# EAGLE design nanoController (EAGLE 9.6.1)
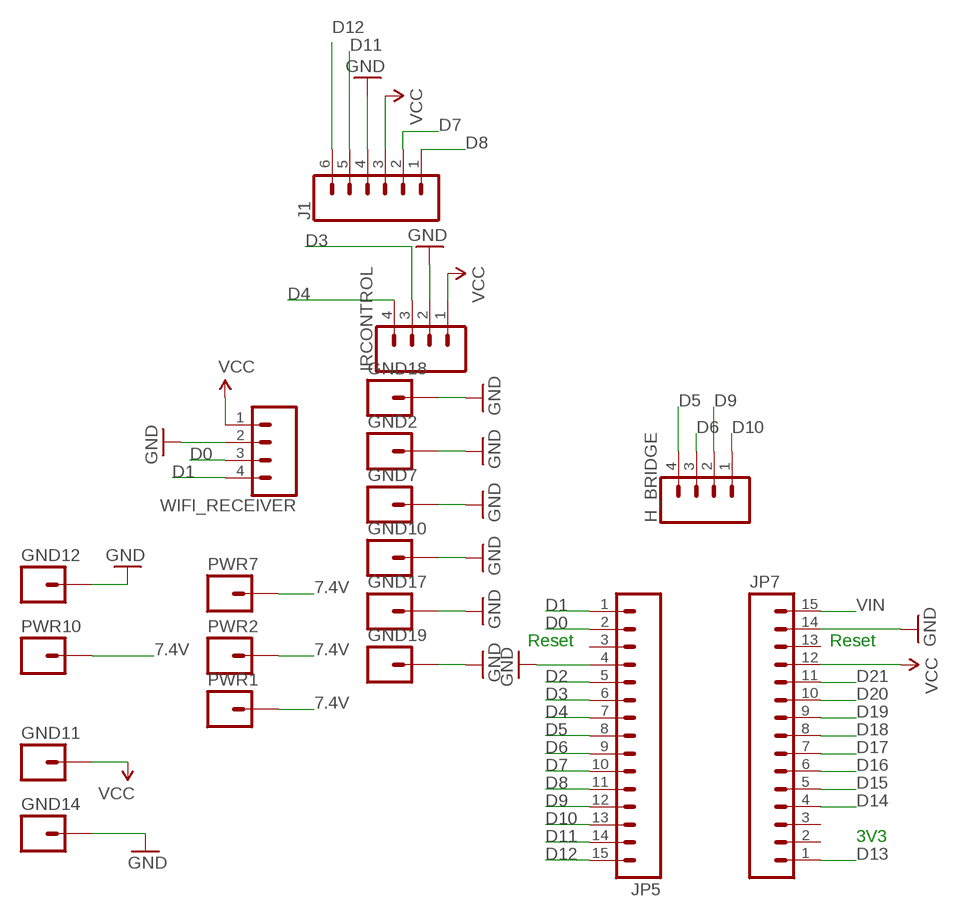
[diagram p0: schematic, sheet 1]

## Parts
GND2  M01PTH_LONGPAD  [1X01_LONGPAD]
GND7  M01PTH_LONGPAD  [1X01_LONGPAD]
GND10  M01PTH_LONGPAD  [1X01_LONGPAD]
GND11  M01PTH_LONGPAD  [1X01_LONGPAD]
GND12  M01PTH_LONGPAD  [1X01_LONGPAD]
GND14  M01PTH_LONGPAD  [1X01_LONGPAD]
GND17  M01PTH_LONGPAD  [1X01_LONGPAD]
GND18  M01PTH_LONGPAD  [1X01_LONGPAD]
GND19  M01PTH_LONGPAD  [1X01_LONGPAD]
H_BRIDGE  CONN_04LONGPADS  [1X04_LONGPADS]
IRCONTROL  CONN_04LONGPADS  [1X04_LONGPADS]
J1  CONN_06SILK_FEMALE_PTH  [1X06]
JP5  M15  [1X15]
JP7  M15  [1X15]
PWR1  M01PTH_LONGPAD  [1X01_LONGPAD]
PWR2  M01PTH_LONGPAD  [1X01_LONGPAD]
PWR7  M01PTH_LONGPAD  [1X01_LONGPAD]
PWR10  M01PTH_LONGPAD  [1X01_LONGPAD]
WIFI_RECEIVER  CONN_04LONGPADS  [1X04_LONGPADS]

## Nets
7.4V: PWR1.1 PWR2.1 PWR7.1 PWR10.1
D0: JP5.2 WIFI_RECEIVER.3
D1: JP5.1 WIFI_RECEIVER.4
D2: JP5.5
D3: IRCONTROL.3 JP5.6
D4: IRCONTROL.4 JP5.7
D5: H_BRIDGE.4 JP5.8
D6: H_BRIDGE.3 JP5.9
D7: J1.2 JP5.10
D8: J1.1 JP5.11
D9: H_BRIDGE.2 JP5.12
D10: H_BRIDGE.1 JP5.13
D11: J1.5 JP5.14
D12: J1.6 JP5.15
D13: JP7.1
D14: JP7.4
D15: JP7.5
D16: JP7.6
D17: JP7.7
D18: JP7.8
D19: JP7.9
D20: JP7.10
D21: JP7.11
GND [gnd]: GND2.1 GND7.1 GND10.1 GND12.1 GND14.1 GND17.1 GND18.1 GND19.1 IRCONTROL.2 J1.4 JP5.4 JP7.14 WIFI_RECEIVER.2
VCC: GND11.1 IRCONTROL.1 J1.3 JP7.12 WIFI_RECEIVER.1
VIN: JP7.15
Unconnected: JP5.3 JP7.2 JP7.3 JP7.13

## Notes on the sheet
- Reset | Reset
- 3V3

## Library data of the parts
GND2 GND7 GND10-GND12 GND14 GND17-GND19 PWR1 PWR2 PWR7 PWR10 = SparkFun-Connectors:M01: Header 1
H_BRIDGE IRCONTROL WIFI_RECEIVER = SparkFun-Connectors:CONN_04: Multi connection point. Often used as Generic Header-pin footprint for 0.1 inch spaced/style header connections On any of the 0.1 inch spaced packages, you can populate with these: Break Away Headers - Straight (PRT-00116) Break Away Male Headers - Right Angle (PRT-00553) Female Headers (PRT-00115)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; PROD_ID: CONN-09696
J1 = SparkFun-Connectors:CONN_06: Multi connection point. Often used as Generic Header-pin footprint for 0.1 inch spaced/style header connections On any of the 0.1 inch spaced packages, you can populate with these: Break Away Headers - Straight (PRT-00116) Break Away Male Headers - Right Angle (PRT-00553) Female Headers (PRT-00115)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; PROD_ID: CONN-08437
JP5 JP7 = SparkFun-Connectors:M15: Header 15 Standard 15-pin 0.1" header. Use with straight break away headers (SKU : PRT-00116), right angle break away headers (PRT-00553), swiss pins (PRT-00743), machine pins (PRT-00117), and female headers (PRT-00115).

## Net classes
0 default: width 0.254 mm, clearance 0.254 mm
1 power: width 0.61 mm, drill 0.711 mm, clearance 0.33 mm
2 gnd: width 0.305 mm, drill 0.711 mm, clearance 0.254 mm
3 usbvcc: width 0.508 mm, drill 0.711 mm, clearance 0.254 mm
4 aref: width 0.406 mm

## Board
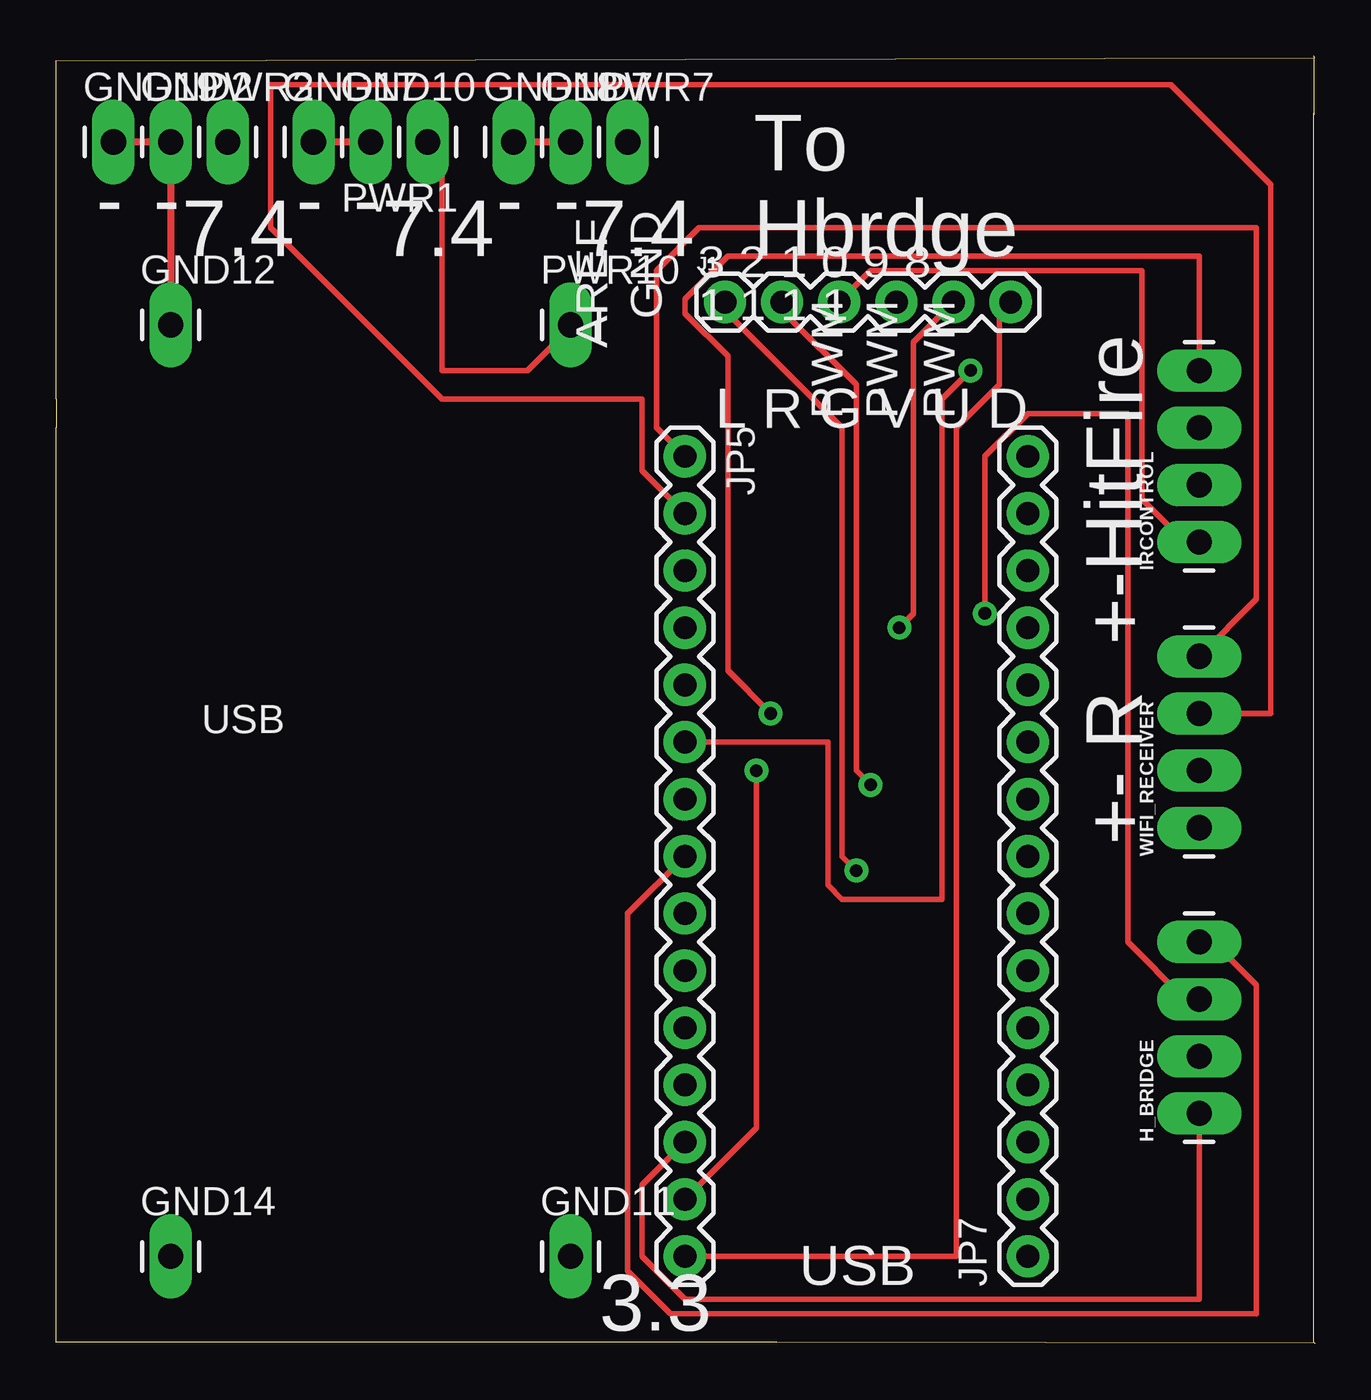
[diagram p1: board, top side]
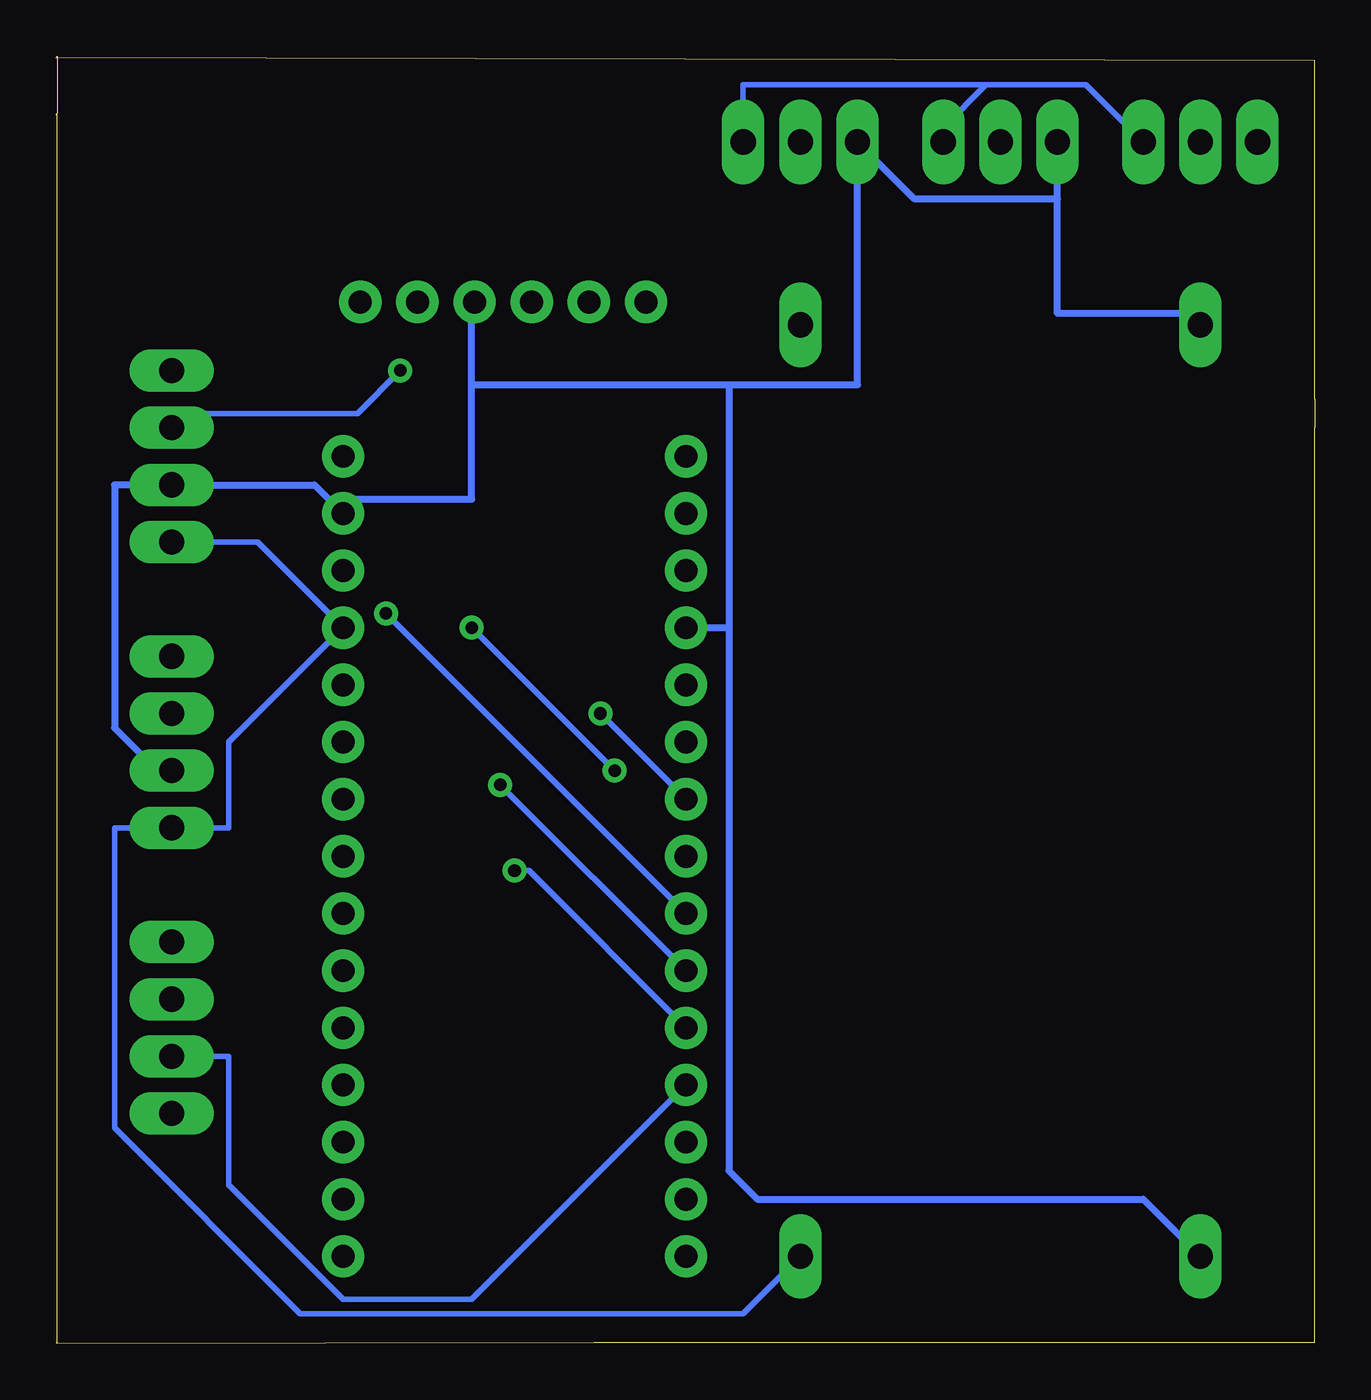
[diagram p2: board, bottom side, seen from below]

Size 55.93 x 57.2 mm. Coordinates in mm from the lower left corner, seen from the top.
Outline: 55.88,54.66 55.88,57.2 55.93,57.12 0,57 0,41.96 0,40.69 0,0.05 32.03,0.05 55.93,0 55.88,0.05 55.88,54.66
Outline: 55.93,54.61 55.88,54.66
Copper layers (1*16): Top 0.035mm / dielectric 1.5mm / Bottom 0.035mm
Design rules "default": minimum track width 10mil, minimum drill 22mil, track to track 10mil, track to pad 10mil, pad to pad 10mil, via to via 16mil, smd to smd 8mil, copper to edge 30mil, drill to drill 12mil, minimum pad ring 10mil, minimum via ring 10mil, stop-mask expansion 4mil, vias tented up to drill 0mil, thermal gap 10mil
vRestrict: area 25.4,45.5 to 27.1,49.2; area 33.4,41.1 to 34.9,44.6; area 35.9,41.1 to 37.5,44.6; area 38.5,41.1 to 40,44.6; area 42.5,38.7 to 43.1,38.9

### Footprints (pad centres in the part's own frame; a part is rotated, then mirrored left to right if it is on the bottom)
1X01_LONGPAD = drill 1.118 pad 1.88 long: 1 0,0
1X04_LONGPADS = drill 1.118 pad 1.88 long: 1 0,0; 2 2.54,0; 3 5.08,0; 4 7.62,0
1X06 = drill 1.016 pad 1.88: 1 0,0; 2 2.54,0; 3 5.08,0; 4 7.62,0; 5 10.16,0; 6 12.7,0
1X15 = drill 1.016 pad 1.88: 1 0,0; 2 2.54,0; 3 5.08,0; 4 7.62,0; 5 10.16,0; 6 12.7,0; 7 15.24,0; 8 17.78,0; 9 20.32,0; 10 22.86,0; 11 25.4,0; 12 27.94,0; 13 30.48,0; 14 33.02,0; 15 35.56,0

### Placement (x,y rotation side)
GND2  5.08,53.39 0 top
GND7  22.86,53.39 0 top
GND10  13.97,53.39 0 top
GND11  22.86,3.86 0 top
GND12  5.08,45.26 0 top
GND14  5.08,3.86 0 top
GND17  11.43,53.39 0 top
GND18  20.32,53.39 0 top
GND19  2.54,53.39 0 top
H_BRIDGE  50.8,10.21 90 top
IRCONTROL  50.8,35.61 90 top
J1  29.72,46.28 0 top
JP5  27.94,39.42 270 top
JP7  43.18,3.86 90 top
PWR1  16.51,53.39 180 top
PWR2  7.62,53.39 0 top
PWR7  25.4,53.39 0 top
PWR10  22.86,45.26 0 top
WIFI_RECEIVER  50.8,22.91 90 top

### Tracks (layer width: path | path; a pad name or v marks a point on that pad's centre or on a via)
7.4V
  Top 0.254: PWR1.1 17.14,52.76 17.14,43.23 20.95,43.23 22.86,45.14 PWR10.1
  Bottom 0.254: PWR2.1 10.16,55.93 14.61,55.93 | 14.61,55.93 16.51,54.03 PWR1.1 | PWR7.1 25.4,55.93 14.61,55.93
D0
  Top 0.254: WIFI_RECEIVER.3 53.98,27.99 53.98,51.49 49.53,55.93 9.53,55.93 9.53,49.58 17.14,41.96 26.04,41.96 26.04,38.79 JP5.2
D1
  Top 0.254: JP5.1 26.67,40.69 26.67,47.68 28.57,49.58 53.34,49.58 53.34,33.07 WIFI_RECEIVER.4
D3  (via drill 0.56)
  Top 0.254: JP5.6 34.29,26.72 34.29,20.37 34.92,19.74 39.37,19.74 39.37,41.96 v40.64,43.23
  Bottom 0.254: v40.64,43.23 42.55,41.33 50.16,41.33 IRCONTROL.3
D4  (via drill 0.56)
  Top 0.254: v31.75,27.99 29.84,29.9 29.84,43.87 27.94,45.77 27.94,46.41 29.84,48.31 50.8,48.31 IRCONTROL.4
  Bottom 0.254: v31.75,27.99 JP5.7
D5
  Top 0.254: JP5.8 25.4,19.1 25.4,3.23 27.3,1.32 53.34,1.32 53.34,15.93 51.44,17.83 H_BRIDGE.4
D6  (via drill 0.56)
  Top 0.254: v41.27,32.44 41.27,39.42 43.18,41.33 47.62,41.33 47.62,17.83 50.16,15.29 H_BRIDGE.3
  Bottom 0.254: v41.27,32.44 JP5.9
D7  (via drill 0.56)
  Top 0.254: v36.2,24.82 35.56,25.45 35.56,42.6 32.38,45.77 J1.2
  Bottom 0.254: v36.2,24.82 JP5.10
D8  (via drill 0.56)
  Top 0.254: v35.56,21.01 34.92,21.64 34.92,40.69 29.84,45.77 J1.1
  Bottom 0.254: JP5.11 34.92,21.01 v35.56,21.01
D9
  Bottom 0.254: JP5.12 37.47,1.96 43.18,1.96 48.26,7.04 48.26,12.75 H_BRIDGE.2
D10
  Top 0.254: JP5.13 26.04,7.04 26.04,3.86 27.94,1.96 50.8,1.96 H_BRIDGE.1
D11  (via drill 0.56)
  Top 0.254: JP5.14 31.11,9.58 v31.11,25.45 | v37.47,31.8 38.1,32.44 38.1,44.5 J1.5
  Bottom 0.254: v37.47,31.8 v31.11,25.45
D12
  Top 0.254: JP5.15 40.01,3.86 40.01,40.69 41.91,42.6 41.91,45.77 J1.6
GND
  Top 0.305: GND7.1 GND18.1 | GND10.1 GND17.1 | GND12.1 GND2.1 GND19.1
  Bottom 0.305: GND14.1 7.62,6.4 24.77,6.4 26.04,7.67 26.04,31.8 | JP5.4 26.04,31.8 | 11.43,50.85 11.43,45.77 5.08,45.77 GND12.1 | 11.43,50.85 GND17.1 | 11.43,50.85 17.78,50.85 GND18.1 20.32,42.6 26.04,42.6 | WIFI_RECEIVER.2 51.44,26.09 52.07,26.09 53.34,27.36 53.34,38.15 IRCONTROL.2 44.45,38.15 43.81,37.52 | 37.47,42.6 37.47,37.52 43.81,37.52 | 37.47,42.6 37.47,45.77 J1.4 | 43.81,37.52 JP7.14 | 37.47,42.6 26.04,42.6 | 26.04,42.6 26.04,31.8
VCC
  Top 0.254: J1.3 36.2,47.68 48.26,47.68 48.26,37.52 50.16,35.61 IRCONTROL.1
  Bottom 0.254: IRCONTROL.1 46.99,35.61 JP7.12 48.26,26.72 48.26,22.91 WIFI_RECEIVER.1 53.34,22.91 53.34,9.58 45.09,1.32 25.4,1.32 GND11.1

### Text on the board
tNames: 3 2 1 0 9 8 | GND | 1 1 1 1 | AREF | PWM | PWM | PWM | USB
Reference: C8 | C2 | R11 | C4 | C5
_tsilk: - | - | - | - | - | - | 7.4 | 7.4 | 7.4 | To / Hbrdge | L R G V U D | +-HitFire | +- R | USB | 3.3

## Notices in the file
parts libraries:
SparkFun-Connectors: Licensing: Creative Commons ShareAlike 4.0 International - https://creativecommons.org/licenses/by-sa/4.0
